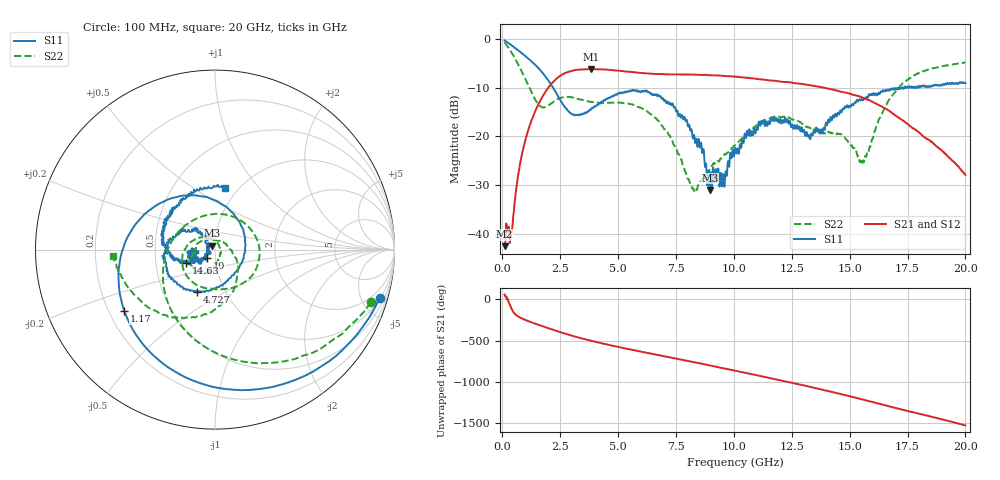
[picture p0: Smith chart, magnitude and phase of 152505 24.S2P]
!  2-Port S-parameters saved by WinCal
! VAR MeasName=S-Parameters (CALIBRATED_DATA) read from VNA (N5230C)
! VAR MeasDate=4/10/2015 9:30:45 AM
! VAR NAME=152505 24
! VAR FILENAME=152505 24.S2P
! VAR DATE=4/10/2015 9:30:45 AM
! VAR PHYS_PORTS=1,2
# Hz S DB R 50
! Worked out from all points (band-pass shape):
!   801 points, 100 MHz to 20 GHz, reference 50 ohm
!   highest |S21| = -6.24 dB at 3.831 GHz (marker M1); lowest = -42.4 dB at 100 MHz (marker M2)
!   |S21| within 3 dB of the highest: 2.121 GHz to 12.9 GHz (10.78 GHz wide, 144 % of centre)
!   lowest |S11| = -30.9 dB at 8.956 GHz (marker M3), VSWR 1.06, Z = 48.2 + j2.16 ohm
!   |S11| at or under -10 dB: 2.187 GHz to 17.26 GHz (15.08 GHz wide, 155 % of centre); 17.28877 GHz to 17.35704 GHz (68.27 MHz wide, 0.394 % of centre); 17.41191 GHz to 17.45157 GHz (39.65 MHz wide, 0.227 % of centre)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
!   |S22| runs from -31.3 to -0.8 dB; largest |S21 - S12| = 0.0062
!   S11 on the Smith chart (normalised r, x): 100 MHz: 1.06, -6.80; 1.17 GHz: 0.26, -0.29; 4.727 GHz: 0.74, -0.37; 10 GHz: 0.91, -0.08; 14.63 GHz: 0.71, -0.11; 20 GHz: 0.87, +0.68
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1e8  -0.38 -16.4  -42.43 57.2  -42.47 58.2  -0.76 -18.8
3.985e8  -1.36 -57.5  -39.64 -114.3  -39.71 -113.9  -2.84 -60.3
5.72625e8  -1.97 -79.4  -31.77 175.6  -31.79 176.0  -4.26 -82.2
1.169625e9  -4.28 -145.7  -17.98 90.2  -17.95 90.3  -10.05 -157.1
2.065125e9  -9.08 121.3  -9.56 2.8  -9.55 2.7  -13.41 54.0
2.687e9  -13.85 46.4  -7.09 -53.8  -7.13 -53.8  -11.97 -14.9
3.43325e9  -15.53 -41.9  -6.32 -113.5  -6.32 -113.3  -12.53 -61.1
3.83125e9  -14.52 -70.5  -6.24 -141.5  -6.25 -141.5  -12.96 -77.0
4.72675e9  -11.89 -113.3  -6.44 160.3  -6.43 160.5  -13.09 -107.0
5.672e9  -10.67 -151.8  -6.85 104.4  -6.83 104.2  -13.57 -145.0
6.741625e9  -11.48 168.2  -7.25 44.7  -7.22 44.3  -16.76 163.7
8.283875e9  -19.69 128.0  -7.37 -41.2  -7.39 -41.2  -31.10 26.8
8.9555e9  -30.93 128.0  -7.49 -79.9  -7.50 -79.7  -26.85 -50.7
1.000025e10  -24.07 -134.9  -7.76 -140.5  -7.78 -140.3  -21.94 -81.0
1.005e10  -22.34 -138.9  -7.79 -143.5  -7.80 -143.6  -21.81 -80.9
1.189075e10  -16.46 -167.0  -8.68 107.8  -8.68 107.7  -15.99 -134.9
1.338325e10  -19.73 -168.1  -9.62 15.2  -9.56 15.3  -18.36 -170.7
1.4627e10  -15.00 -155.8  -10.85 -66.4  -10.86 -66.9  -19.54 162.5
1.554738e10  -12.40 -167.1  -12.03 -130.8  -12.10 -131.6  -25.60 66.6
1.669162e10  -10.61 169.4  -14.72 146.5  -14.82 145.1  -12.58 -61.5
1.798512e10  -9.64 139.1  -19.10 56.7  -19.32 56.7  -7.01 -121.8
2e10  -9.12 81.0  -27.87 -85.8  -27.87 -84.6  -4.87 -176.5
